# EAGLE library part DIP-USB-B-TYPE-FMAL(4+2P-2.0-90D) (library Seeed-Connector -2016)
320010018
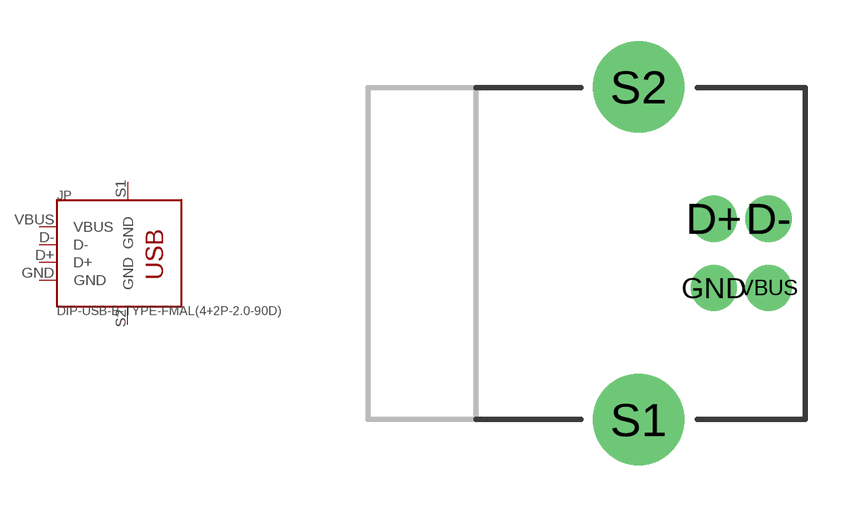
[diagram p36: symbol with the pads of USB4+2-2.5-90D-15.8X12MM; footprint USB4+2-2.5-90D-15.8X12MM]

Designator prefix JP

## DIP-USB-B-TYPE-FMAL(4+2P-2.0-90D)  [USB4+2-2.5-90D-15.8X12MM]
D+  D+
D-  D-
GND  GND
S1  GND
S2  GND
VBUS  VBUS

## Footprint USB4+2-2.5-90D-15.8X12MM (pad centres in mm)
USB Series B Hole Mounted
drill 0.914 pad 1.676: D+ 0,1.25; D- 1.981,1.25; GND 0,-1.25; VBUS 1.981,-1.25
drill 2.286: S1 -2.718,-6.02; S2 -2.718,6.02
